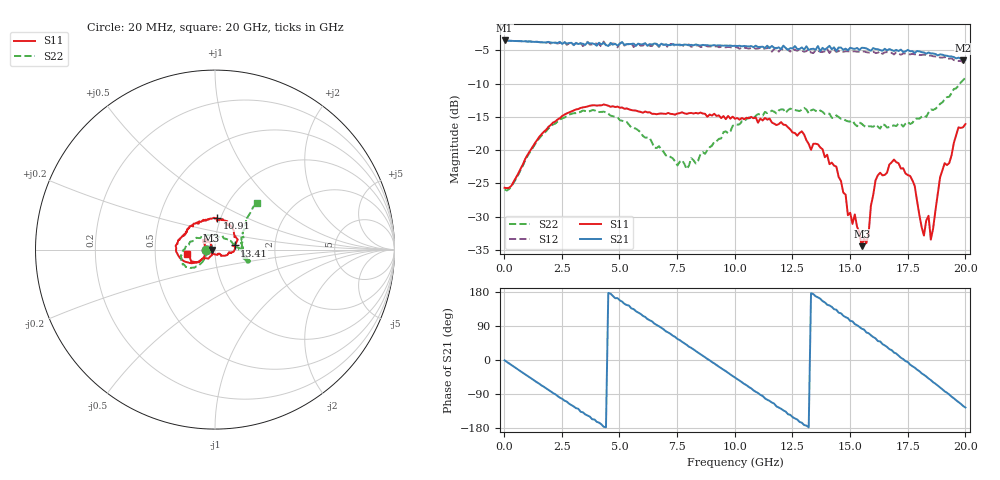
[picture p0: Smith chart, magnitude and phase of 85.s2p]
!Agilent Technologies,N5230A,US43500223,A.07.50.48
!Agilent N5230A: A.07.50.48
!Date: Wednesday, September 16, 2015 17:30:06
!Correction: S11(Full 2 Port(1,2))
!S21(Full 2 Port(1,2))
!S12(Full 2 Port(1,2))
!S22(Full 2 Port(1,2))
!S2P File: Measurements: S11, S21, S12, S22:
# Hz S  dB  R 50
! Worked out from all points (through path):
!   201 points, 20 MHz to 20 GHz, reference 50 ohm
!   highest |S21| = -3.52 dB at 20 MHz (marker M1); lowest = -6.5 dB at 19.9 GHz (marker M2)
!   group delay of S21, straight-line fit = 116 ps
!   lowest |S11| = -34.4 dB at 15.5 GHz (marker M3), VSWR 1.04, Z = 48.2 - j0.233 ohm
!   |S11| at or under -10 dB: start of sweep to end of sweep
!   |S22| runs from -26.1 to -9.1 dB; largest |S21 - S12| = 0.08
!   S11 on the Smith chart (normalised r, x): 20 MHz: 0.90, -0.00; 10.91 GHz: 0.96, +0.35; 13.41 GHz: 1.24, +0.06; 20 GHz: 0.73, -0.04
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2e7  -25.66 -179.0  -3.52 -1.0  -3.53 -1.0  -25.92 179.5
1.9181e9  -16.52 -149.4  -3.74 -78.9  -3.76 -79.9  -16.75 -138.3
3.4166e9  -13.58 -172.4  -4.02 -138.2  -4.37 -138.9  -14.05 -155.1
4.3157e9  -13.14 174.8  -3.91 -176.3  -3.69 -175.5  -14.23 -170.1
5.1149e9  -13.59 164.5  -3.76 154.1  -3.80 152.3  -15.59 176.1
6.7133e9  -14.53 151.2  -4.36 89.1  -4.51 86.4  -19.41 133.3
8.4116e9  -14.50 138.9  -4.23 19.5  -4.27 15.8  -21.58 47.0
1.001e10  -15.28 111.7  -4.33 -46.2  -4.47 -49.0  -16.17 -6.9
1.09091e10  -15.08 86.6  -4.31 -83.9  -4.77 -86.8  -14.85 -15.2
1.22078e10  -16.22 51.9  -4.68 -136.1  -4.67 -141.4  -14.40 -17.0
1.34066e10  -19.06 12.1  -4.77 173.8  -5.41 170.9  -13.89 -21.0
1.44056e10  -22.49 -23.9  -5.12 132.6  -5.25 127.1  -14.78 -17.4
1.55045e10  -34.43 -172.7  -4.62 82.5  -5.21 80.2  -16.04 -6.5
1.58042e10  -32.51 167.9  -4.91 70.6  -5.35 66.8  -16.41 -4.7
1.61039e10  -24.53 159.7  -4.82 57.1  -5.41 54.1  -16.18 1.6
1.67033e10  -22.17 147.5  -4.82 28.6  -5.37 26.4  -16.53 10.0
1.76024e10  -23.88 138.5  -5.14 -12.2  -5.61 -13.3  -16.08 19.7
1.82018e10  -32.84 158.9  -5.33 -38.9  -5.66 -42.1  -14.81 28.8
1.85015e10  -33.45 -165.2  -5.47 -53.0  -5.81 -56.8  -13.90 34.7
1.89011e10  -24.13 -126.1  -5.61 -72.4  -6.10 -75.6  -13.06 38.0
1.99001e10  -16.57 -165.0  -6.51 -121.2  -6.83 -125.9  -9.47 47.5
2e10  -16.09 -170.7  -6.42 -125.3  -6.97 -131.7  -9.11 48.0
